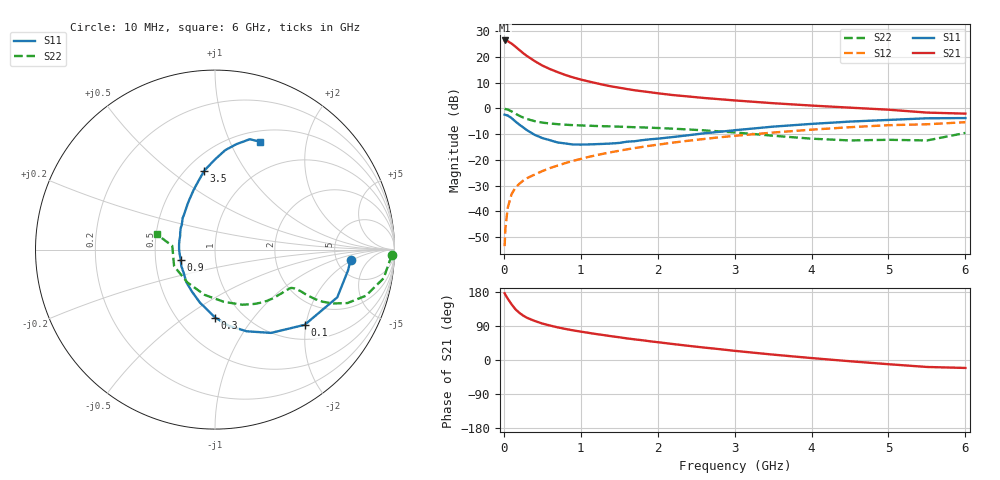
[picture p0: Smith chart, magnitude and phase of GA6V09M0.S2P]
! Infineon Technologies  Discrete & RF Semiconductors
! BF775
! Si NPN RF Bipolar Junction Transistor in SOT23
! VCE = 6 V  IC = 9 mA
! Common Emitter S-Parameters:  May  1996
# GHz  S  MA  R  50
!  f  S11  S21  S12  S22
! GHz  MAG  ANG  MAG  ANG  MAG  ANG  MAG  ANG
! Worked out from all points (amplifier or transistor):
!   36 points, 10 MHz to 6 GHz, reference 50 ohm
!   highest |S21| = 26.5 dB at 10 MHz (marker M1)
!   |S21| within 3 dB of that: start of sweep to 174.1 MHz
!   unconditionally stable (mu >= 1): 645.7 MHz to 2.974 GHz
!   at 250 MHz: K = 0.64, MSG = 24.8 dB, |S12| = -28.1 dB
!   at 1.4 GHz: K = 1.10, MAG = 10.8 dB, |S12| = -17.0 dB
!   at 6 GHz: K = 0.91, MSG = 1.7 dB, |S12| = -5.3 dB
!   S11 on the Smith chart (normalised r, x): 10 MHz: 6.79, -1.77; 100 MHz: 1.35, -1.97; 300 MHz: 0.75, -0.66; 900 MHz: 0.68, -0.08; 3.5 GHz: 0.61, +0.67; 6 GHz: 0.63, +1.31
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0.01  0.7579 -4.2  21.04 176.1  0.0021 89.0  0.9888 -1.8
0.02  0.7502 -8.8  20.96 172.2  0.0046 84.7  0.9743 -3.9
0.05  0.7315 -21.3  20.45 162.1  0.0116 79.2  0.9534 -9.6
0.1  0.6521 -40.0  18.3 147.1  0.0215 71.8  0.8792 -17.0
0.15  0.5592 -56.1  15.98 134.0  0.0289 66.3  0.7953 -22.0
0.2  0.4877 -68.9  13.81 124.8  0.0341 63.8  0.7236 -24.5
0.25  0.4307 -79.9  11.95 117.4  0.0394 62.3  0.6679 -25.8
0.3  0.3788 -89.8  10.5 111.5  0.0441 62.1  0.6259 -26.3
0.4  0.3073 -105.8  8.37 103.1  0.0518 62.0  0.5674 -26.3
0.5  0.266 -119.2  6.849 96.2  0.0606 63.2  0.5311 -25.9
0.6  0.2414 -131.6  5.84 90.9  0.0694 63.8  0.5105 -25.9
0.7  0.2182 -142.9  5.092 86.1  0.0776 64.1  0.4955 -26.0
0.9  0.1992 -163.4  4.02 78.2  0.0959 64.7  0.4743 -26.8
1.1  0.2001 179.3  3.36 71.7  0.1142 64.7  0.4629 -28.7
1.3  0.2052 165.0  2.874 65.7  0.1325 63.6  0.452 -30.8
1.6  0.2257 147.9  2.388 57.0  0.1603 61.8  0.4375 -34.9
2.2  0.2786 125.5  1.823 42.1  0.217 57.1  0.4049 -45.1
3  0.3773 105.8  1.435 24.2  0.2938 48.8  0.3422 -63.8
3.5  0.4436 97.8  1.267 14.2  0.3403 42.9  0.2952 -80.3
4.5  0.5564 84.2  1.038 -3.3  0.4327 30.4  0.2391 -130.0
5.5  0.645 72.5  0.832 -18.4  0.4931 15.4  0.2388 175.0
6  0.651 67.2  0.794 -21.0  0.5411 11.3  0.3347 165.4
